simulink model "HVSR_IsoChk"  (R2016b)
settings: Solver=VariableStepAuto  StartTime=0.0  StopTime=10.0  RelTol=1e-3
undefined symbols (not defined in the file or in its folder): bin2dec, enmActv, enmBmsMode, enmCctErr, enmSWSta, HVSR_bIsoResShieldCal, HVSR_bSw1EnaByMnl_C, HVSR_bSw2EnaByMnl_C, HVSR_bSw3EnaByMnl_C, HVSR_bSwEnaByMnl_C, HVSR_bVldEnaByMnl_C, HVSR_cntIsoChkCnfDiag_C, HVSR_cntIsoChkCnfLv1Diag_C, HVSR_cntIsoChkDiag_CW, HVSR_cntPwrDown_C, HVSR_cofPosVoltfilter_C, HVSR_cofResGain_C, HVSR_deltInsRes_C, HVSR_InsResCtrlSw_C, HVSR_kSlopeVal_C, HVSR_numBgnTimeCnt_C, HVSR_numCycleTimeCnt_C, HVSR_numIsoCnst_C, HVSR_numSlopeCnfrm_C, HVSR_ResFirstCtrlSw_C, HVSR_resIsoFaultLvl1Thres_C, HVSR_resIsoFaultLvl2Thres_C, HVSR_ResR1_C, HVSR_ResR2_C, HVSR_ResR3_C, HVSR_resRstnUpLim_C, HVSR_rIsoCnfHysDiag_C, HVSR_rIsoCnfHysLv1Diag_C, HVSR_stBMSModeLvl_C, HVSR_tiChkFilteTime_C, HVSR_tiIsoChkCycl_T, HVSR_tiIsoChkDebounce_C, HVSR_tiIsoVldChkDebounce_C, HVSR_tiTaskTime_C, HVSR_tiVoltDiffThres_C, HVSR_uBattVoltRngHi_C, HVSR_uBattVoltRngLo_C, HVSR_uIsoKVoltThres_C, HVSR_uIsoPosVoltFilter_C, HVSR_uIsoVoltThres_C
libraries: simulink x78
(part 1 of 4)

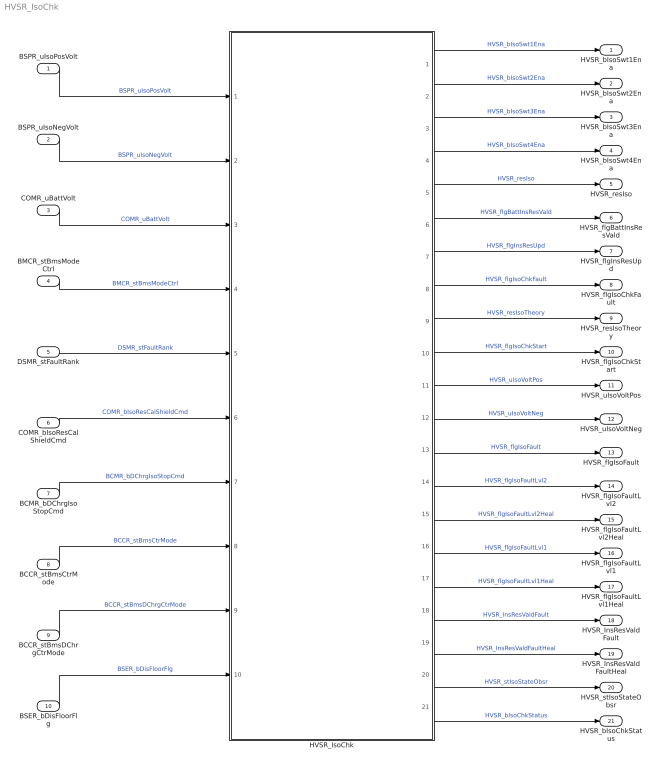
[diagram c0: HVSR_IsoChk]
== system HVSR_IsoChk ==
  BSPR_uIsoPosVolt : Inport  Description=Power battery postive to case voltage
  BSPR_uIsoNegVolt : Inport  Description=Power battery negative to case voltage  Port=2
  COMR_uBattVolt : Inport  Description=Battery pack total voltage  Port=3
  BMCR_stBmsModeCtrl : Inport  Port=4
  DSMR_stFaultRank : Inport  Port=5
  COMR_bIsoResCalShieldCmd : Inport  Port=6
  BCMR_bDChrgIsoStopCmd : Inport  Port=7
  BCCR_stBmsCtrMode : Inport  Port=8
  BCCR_stBmsDChrgCtrMode : Inport  Port=9
  BSER_bDisFloorFlg : Inport  Port=10
  HVSR_IsoChk : Subsystem  Description=Battery pack insulation detection module
  HVSR_bIsoSwt1Ena : Outport  Description=Insulation detection positive relay control command
  HVSR_bIsoSwt2Ena : Outport  Description=Insulation detection positive relay control command  Port=2
  HVSR_bIsoSwt3Ena : Outport  Description=Insulation detection positive relay control command  Port=3
  HVSR_bIsoSwt4Ena : Outport  Description=Insulation detection positive relay control command  Port=4
  HVSR_resIso : Outport  Description=Insulation detection resistance validity flag  Port=5
  HVSR_flgBattInsResVald : Outport  Description=Insulation detection resistance validity flag  Port=6
  HVSR_flgInsResUpd : Outport  Description=Insulation detection resistance pass flag  Port=7
  HVSR_flgIsoChkFault : Outport  Description=Insulation detection resistance pass flag  Port=8
  HVSR_resIsoTheory : Outport  Description=Insulation detection resistance pass flag  Port=9
  HVSR_flgIsoChkStart : Outport  Port=10
  HVSR_uIsoVoltPos : Outport  Port=11
  HVSR_uIsoVoltNeg : Outport  Port=12
  HVSR_flgIsoFault : Outport  Description=Insulation detection resistance pass flag  Port=13
  HVSR_flgIsoFaultLvl2 : Outport  Port=14
  HVSR_flgIsoFaultLvl2Heal : Outport  Port=15
  HVSR_flgIsoFaultLvl1 : Outport  Port=16
  HVSR_flgIsoFaultLvl1Heal : Outport  Port=17
  HVSR_InsResValdFault : Outport  Port=18
  HVSR_InsResValdFaultHeal : Outport  Port=19
  HVSR_stIsoStateObsr : Outport  Port=20
  HVSR_bIsoChkStatus : Outport  Port=21
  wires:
  BSPR_uIsoPosVolt/1 -> HVSR_IsoChk/1(BSPR_uIsoPosVolt)  "BSPR_uIsoPosVolt"
  COMR_uBattVolt/1 -> HVSR_IsoChk/3(BSPR_uBattVolt)  "COMR_uBattVolt"
  HVSR_IsoChk/1(HVSR_bIsoSwt1Ena) -> HVSR_bIsoSwt1Ena/1  "HVSR_bIsoSwt1Ena"
  HVSR_IsoChk/2(HVSR_bIsoSwt2Ena) -> HVSR_bIsoSwt2Ena/1  "HVSR_bIsoSwt2Ena"
  HVSR_IsoChk/3(HVSR_bIsoSwt3Ena) -> HVSR_bIsoSwt3Ena/1  "HVSR_bIsoSwt3Ena"
  HVSR_IsoChk/6(HVSR_flgBattInsResVald) -> HVSR_flgBattInsResVald/1  "HVSR_flgBattInsResVald"
  HVSR_IsoChk/13(HVSR_flgIsoFault) -> HVSR_flgIsoFault/1  "HVSR_flgIsoFault"
  HVSR_IsoChk/5(HVSR_resIso) -> HVSR_resIso/1  "HVSR_resIso"
  HVSR_IsoChk/7(HVSR_flgInsResUpd) -> HVSR_flgInsResUpd/1  "HVSR_flgInsResUpd"
  HVSR_IsoChk/8(HVSR_flgIsoChkFault) -> HVSR_flgIsoChkFault/1  "HVSR_flgIsoChkFault"
  HVSR_IsoChk/9(HVSR_resIsoTheory) -> HVSR_resIsoTheory/1  "HVSR_resIsoTheory"
  HVSR_IsoChk/11(HVSR_uIsoVoltPos) -> HVSR_uIsoVoltPos/1  "HVSR_uIsoVoltPos"
  HVSR_IsoChk/10(HVSR_flgIsoChkStart) -> HVSR_flgIsoChkStart/1  "HVSR_flgIsoChkStart"
  DSMR_stFaultRank/1 -> HVSR_IsoChk/5(DSMR_stFaultRank)  "DSMR_stFaultRank"
  BMCR_stBmsModeCtrl/1 -> HVSR_IsoChk/4(BMCR_stBmsModeCtrl)  "BMCR_stBmsModeCtrl"
  HVSR_IsoChk/14(HVSR_flgIsoFaultLvl2) -> HVSR_flgIsoFaultLvl2/1  "HVSR_flgIsoFaultLvl2"
  HVSR_IsoChk/15(HVSR_flgIsoFaultLvl2Heal) -> HVSR_flgIsoFaultLvl2Heal/1  "HVSR_flgIsoFaultLvl2Heal"
  HVSR_IsoChk/16(HVSR_flgIsoFaultLvl1) -> HVSR_flgIsoFaultLvl1/1  "HVSR_flgIsoFaultLvl1"
  HVSR_IsoChk/17(HVSR_flgIsoFaultLvl1Heal) -> HVSR_flgIsoFaultLvl1Heal/1  "HVSR_flgIsoFaultLvl1Heal"
  HVSR_IsoChk/19(HVSR_InsResValdFaultHeal) -> HVSR_InsResValdFaultHeal/1  "HVSR_InsResValdFaultHeal"
  HVSR_IsoChk/18(HVSR_InsResValdFault) -> HVSR_InsResValdFault/1  "HVSR_InsResValdFault"
  COMR_bIsoResCalShieldCmd/1 -> HVSR_IsoChk/6(COMR_bIsoResCalShieldCmd)  "COMR_bIsoResCalShieldCmd"
  BCMR_bDChrgIsoStopCmd/1 -> HVSR_IsoChk/7(BCMR_bDChrgIsoStopCmd)  "BCMR_bDChrgIsoStopCmd"
  HVSR_IsoChk/20(HVSR_stIsoStateObsr) -> HVSR_stIsoStateObsr/1  "HVSR_stIsoStateObsr"
  HVSR_IsoChk/21(HVSR_bIsoChkStatus) -> HVSR_bIsoChkStatus/1  "HVSR_bIsoChkStatus"
  BSPR_uIsoNegVolt/1 -> HVSR_IsoChk/2(BSPR_uIsoNegVolt)  "BSPR_uIsoNegVolt"
  HVSR_IsoChk/4(HVSR_bIsoSwt4Ena) -> HVSR_bIsoSwt4Ena/1  "HVSR_bIsoSwt4Ena"
  HVSR_IsoChk/12(HVSR_uIsoVoltNeg) -> HVSR_uIsoVoltNeg/1  "HVSR_uIsoVoltNeg"
  BCCR_stBmsCtrMode/1 -> HVSR_IsoChk/8(BCCR_stBmsCtrMode)  "BCCR_stBmsCtrMode"
  BCCR_stBmsDChrgCtrMode/1 -> HVSR_IsoChk/9(BCCR_stBmsDChrgCtrMode)  "BCCR_stBmsDChrgCtrMode"
  BSER_bDisFloorFlg/1 -> HVSR_IsoChk/10(BSER_bDisFloorFlg)  "BSER_bDisFloorFlg"

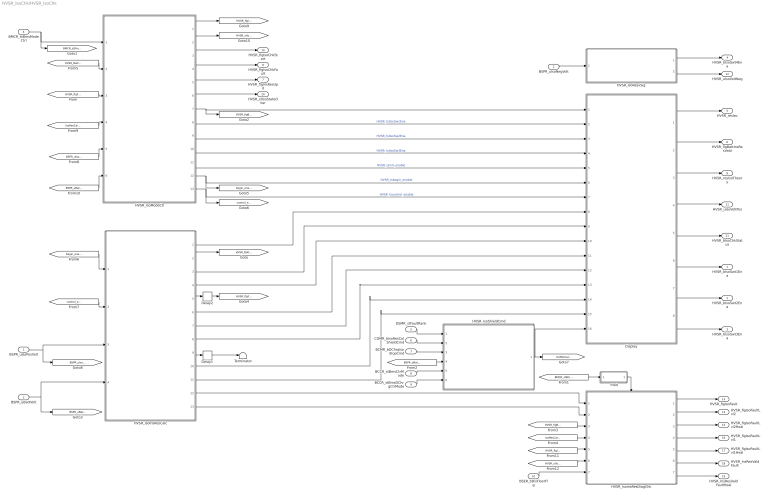
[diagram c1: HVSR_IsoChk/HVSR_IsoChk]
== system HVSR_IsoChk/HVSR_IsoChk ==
  BSPR_uIsoPosVolt : Inport
  BSPR_uIsoNegVolt : Inport  Description=Power battery negative to case voltage  Port=2
  BSPR_uBattVolt : Inport  Port=3
  BMCR_stBmsModeCtrl : Inport  Port=4
  DSMR_stFaultRank : Inport  Port=5
  COMR_bIsoResCalShieldCmd : Inport  Port=6
  BCMR_bDChrgIsoStopCmd : Inport  Port=7
  BCCR_stBmsCtrMode : Inport  Port=8
  BCCR_stBmsDChrgCtrMode : Inport  Port=9
  BSER_bDisFloorFlg : Inport  Port=10
  Delay1 : Delay  DelayLength=1  InitialCondition=0
  Delay2 : Delay  DelayLength=1  InitialCondition=0
  Display : Subsystem  Description=Battery pack insulation detection Display module
  HVSR_IsoInsResCalc : Subsystem  Description=Battery pack insulation detection Control module
  HVSR_IsoInsResDiagChk : Subsystem
  HVSR_IsoModeCtr : Subsystem
  HVSR_IsoResvSig : Subsystem
  HVSR_IsoShieldCmd : Subsystem
  Terminator : Terminator
  mod : Subsystem
  HVSR_bIsoSwt1Ena : Outport
  HVSR_bIsoSwt2Ena : Outport  Port=2
  HVSR_bIsoSwt3Ena : Outport  Port=3
  HVSR_bIsoSwt4Ena : Outport  Port=4
  HVSR_resIso : Outport  Port=5
  HVSR_flgBattInsResVald : Outport  Port=6
  HVSR_flgInsResUpd : Outport  Port=7
  HVSR_flgIsoChkFault : Outport  Port=8
  HVSR_resIsoTheory : Outport  Port=9
  HVSR_flgIsoChkStart : Outport  Port=10
  HVSR_uIsoVoltPos : Outport  Port=11
  HVSR_uIsoVoltNeg : Outport  Port=12
  HVSR_flgIsoFault : Outport  Port=13
  HVSR_flgIsoFaultLvl2 : Outport  Port=14
  HVSR_flgIsoFaultLvl2Heal : Outport  Port=15
  HVSR_flgIsoFaultLvl1 : Outport  Port=16
  HVSR_flgIsoFaultLvl1Heal : Outport  Port=17
  HVSR_InsResValdFault : Outport  Port=18
  HVSR_InsResValdFaultHeal : Outport  Port=19
  HVSR_stIsoStateObsr : Outport  Port=20
  HVSR_bIsoChkStatus : Outport  Port=21
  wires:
  BSPR_uBattVolt/1 -> HVSR_IsoInsResCalc/4(BSPR_uBattVolt), [BSPR_uBattVolt]
  Display/1(HVSR_resIso) -> HVSR_resIso/1
  Display/2(HVSR_flgBattInsResVald) -> HVSR_flgBattInsResVald/1
  Display/3(HVSR_resIsoTheory) -> HVSR_resIsoTheory/1
  Display/4(HVSR_uIsoVoltPos) -> HVSR_uIsoVoltPos/1
  HVSR_IsoInsResCalc/2(HVSR_BattInsResVald) -> [HVSR_BattInsResVald]
  HVSR_IsoInsResDiagChk/1(HVSR_flgIsoFault) -> HVSR_flgIsoFault/1
  HVSR_IsoInsResDiagChk/2(HVSR_flgIsoFaultLvl2) -> HVSR_flgIsoFaultLvl2/1
  HVSR_IsoInsResDiagChk/3(HVSR_flgIsoFaultLvl2Heal) -> HVSR_flgIsoFaultLvl2Heal/1
  HVSR_IsoInsResDiagChk/4(HVSR_flgIsoFaultLvl1) -> HVSR_flgIsoFaultLvl1/1
  HVSR_IsoInsResDiagChk/5(HVSR_flgIsoFaultLvl1Heal) -> HVSR_flgIsoFaultLvl1Heal/1
  BSPR_uIsoPosVolt/1 -> HVSR_IsoInsResCalc/3(BSPR_uIsoPosVolt), [BSPR_uIsoNegVolt]
  HVSR_IsoInsResCalc/5(HVSR_flgFrstRsVlotVld) -> Delay2/1
  Delay2/1 -> [HVSR_flgFrstRsVlotVld]
  mod/1(Out1) -> HVSR_IsoInsResDiagChk/Enable
  HVSR_IsoInsResDiagChk/6(HVSR_InsResValdFault) -> HVSR_InsResValdFault/1
  HVSR_IsoInsResDiagChk/7(HVSR_InsResValdFaultHeal) -> HVSR_InsResValdFaultHeal/1
  Display/5(HVSR_bIsoChkStatus) -> HVSR_bIsoChkStatus/1
  DSMR_stFaultRank/1 -> HVSR_IsoShieldCmd/1(DSMR_stFaultRank)
  COMR_bIsoResCalShieldCmd/1 -> HVSR_IsoShieldCmd/2(COMR_bIsoResCalShieldCmd)
  BCMR_bDChrgIsoStopCmd/1 -> HVSR_IsoShieldCmd/3(BCMR_bDChrgIsoStopCmd)
  HVSR_IsoModeCtr/3(HVSR_flgIsoChkStart) -> HVSR_flgIsoChkStart/1
  HVSR_IsoModeCtr/4(HVSR_flgIsoChkFault) -> HVSR_flgIsoChkFault/1
  HVSR_IsoModeCtr/5(HVSR_flgInsResUpd) -> HVSR_flgInsResUpd/1
  HVSR_IsoModeCtr/6(HVSR_stIsoStateObsr) -> HVSR_stIsoStateObsr/1
  [HVSR_BattInsResVald] -> HVSR_IsoModeCtr/2(HVSR_BattInsResVald)
  [HVSR_flgFrstRsVlotVld] -> HVSR_IsoModeCtr/3(HVSR_flgFrstRsVlotVld)
  [IsoResCalShieldCmd] -> HVSR_IsoModeCtr/4(IsoResCalShieldCmd)
  BSPR_uIsoNegVolt/1 -> HVSR_IsoResvSig/1(BSPR_uIsoNegVolt)
  HVSR_IsoResvSig/1(HVSR_bIsoSwt4Ena) -> HVSR_bIsoSwt4Ena/1
  HVSR_IsoResvSig/2(HVSR_uIsoVoltNeg) -> HVSR_uIsoVoltNeg/1
  HVSR_IsoModeCtr/12(begin_enable) -> [begin_enable], Display/6(begin_enable)  "HVSR_tsbegin_enable"
  HVSR_IsoInsResCalc/1(HVSR_IsoBattInsRes) -> Display/8(HVSR_IsoBattInsRes)
  HVSR_IsoInsResCalc/3(HVSR_IsoInsResTheory) -> Display/9(HVSR_IsoResThry)
  HVSR_IsoInsResCalc/12(flgIsoFaultLvl1) -> HVSR_IsoInsResDiagChk/1(flgIsoFaultLvl1)
  HVSR_IsoInsResCalc/13(flgIsoFaultLvl2) -> HVSR_IsoInsResDiagChk/2(flgIsoFaultLvl2)
  Display/6(HVSR_bIsoSwt1Ena) -> HVSR_bIsoSwt1Ena/1
  Display/8(HVSR_bIsoSwt3Ena) -> HVSR_bIsoSwt3Ena/1
  HVSR_IsoModeCtr/11(init_enable) -> Display/5(init_enable)  "HVSR_tsinit_enable"
  [BMCR_stBmsModeCtrl] -> mod/1(In1)
  [HVSR_flgBattInsResVld] -> HVSR_IsoInsResDiagChk/3(flgBattInsResVald)
  HVSR_IsoModeCtr/7(HVSR_flgBattInsResVld) -> [HVSR_flgBattInsResVld], Display/1(HVSR_IsoResVald)
  HVSR_IsoModeCtr/8(HVSR_IsoSwt1Ena) -> Display/2(bIsoSwt1Ena)  "HVSR_tsIIsoSw1Ena"
  HVSR_IsoModeCtr/9(HVSR_IsoSwt2Ena) -> Display/3(bIsoSwt2Ena)  "HVSR_tsIIsoSw2Ena"
  HVSR_IsoModeCtr/10(HVSR_IsoSwt3Ena) -> Display/4(bIsoSwt3Ena)  "HVSR_tsIIsoSw3Ena"
  [IsoResCalShieldCmd] -> HVSR_IsoInsResDiagChk/4(IsoResCalShield)
  HVSR_IsoShieldCmd/1(HVSR_IsoChieldCmd) -> Display/16(HVSR_IsoChieldCmd), [IsoResCalShieldCmd]
  HVSR_IsoInsResCalc/4("HVSR_uIsoFrstRsVolt ") -> Display/10(HVSR_uIsoFrstRsVolt)
  HVSR_IsoInsResCalc/8(HVSR_uIsoScndRsVolt) -> Display/13(HVSR_uIsoScndRsVolt)
  HVSR_IsoInsResCalc/9(HVSR_flgScndRsVlotVld) -> Delay1/1
  Delay1/1 -> Terminator/1
  HVSR_IsoModeCtr/13(control_enable) -> [control_enable], Display/7(control_enable)  "HVSR_tscontrol_enable"
  HVSR_IsoInsResCalc/7(HVSR_numIsoFrstVal) -> Display/12(HVSR_numIsoFrstVal)
  HVSR_IsoInsResCalc/6(HVSR_uFrstRsVlot) -> Display/11(HVSR_uFrstRsVlot)
  HVSR_IsoInsResCalc/11(HVSR_numIsoScndVal) -> Display/15(HVSR_numIsoScndVal)
  HVSR_IsoInsResCalc/10(HVSR_uScndRsVlot) -> Display/14(HVSR_uScndRsVlot)
  BMCR_stBmsModeCtrl/1 -> [BMCR_stBmsModeCtrl], HVSR_IsoModeCtr/1(BMCR_stBmsModeCtrl)
  Display/7(HVSR_bIsoSwt2Ena) -> HVSR_bIsoSwt2Ena/1
  [begin_enable] -> HVSR_IsoInsResCalc/1(begin_enable)
  [control_enable] -> HVSR_IsoInsResCalc/2(control_enable)
  [BSPR_uBattVolt] -> HVSR_IsoShieldCmd/4(BSPR_uBattVolt)
  BCCR_stBmsCtrMode/1 -> HVSR_IsoShieldCmd/5(BCCR_stBmsCtrMode)
  BCCR_stBmsDChrgCtrMode/1 -> HVSR_IsoShieldCmd/6(BCCR_stBmsDChrgCtrMode)
  [BSPR_uIsoNegVolt] -> HVSR_IsoModeCtr/5(BSPR_uIsoNegVolt)
  [BSPR_uBattVolt] -> HVSR_IsoModeCtr/6(BSPR_uBattVolt)
  HVSR_IsoModeCtr/1(HVSR_flgIsoCctChkOK) -> [HVSR_flgIsoCctChkOK]
  HVSR_IsoModeCtr/2(HVSR_stIsoCctChkErr) -> [HVSR_stIsoCctChkErr]
  [HVSR_flgIsoCctChkOK] -> HVSR_IsoInsResDiagChk/5(HVSR_flgIsoCctChkOK)
  [HVSR_stIsoCctChkErr] -> HVSR_IsoInsResDiagChk/6(HVSR_stIsoCctChkE rr)
  BSER_bDisFloorFlg/1 -> HVSR_IsoInsResDiagChk/7(BSER_bDisFloorFlg)

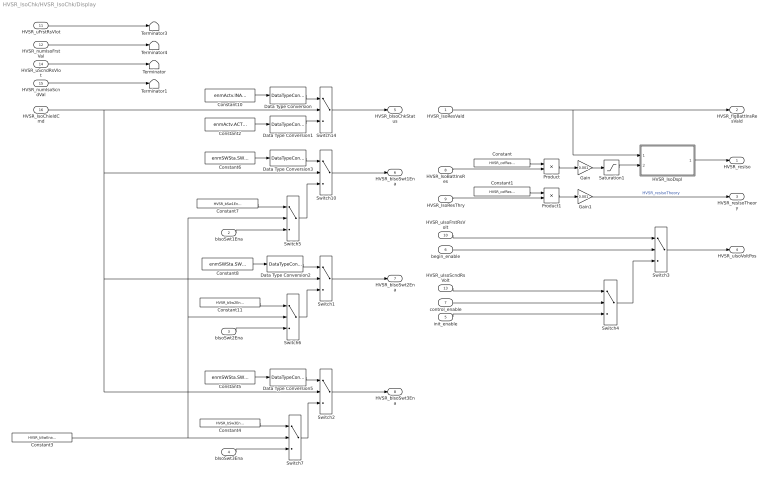
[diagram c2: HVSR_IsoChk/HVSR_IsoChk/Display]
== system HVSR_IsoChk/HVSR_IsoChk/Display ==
  HVSR_IsoResVald : Inport
  bIsoSwt1Ena : Inport  Port=2
  bIsoSwt2Ena : Inport  Port=3
  bIsoSwt3Ena : Inport  Port=4
  init_enable : Inport  Port=5
  begin_enable : Inport  Port=6
  control_enable : Inport  Port=7
  HVSR_IsoBattInsRes : Inport  Port=8
  HVSR_IsoResThry : Inport  Port=9
  HVSR_uIsoFrstRsVolt : Inport  Port=10
  HVSR_uFrstRsVlot : Inport  Port=11
  HVSR_numIsoFrstVal : Inport  Port=12
  HVSR_uIsoScndRsVolt : Inport  Port=13
  HVSR_uScndRsVlot : Inport  Port=14
  HVSR_numIsoScndVal : Inport  Port=15
  HVSR_IsoChieldCmd : Inport  Port=16
  Constant : Constant  Value=HVSR_cofResGain_C
  Constant1 : Constant  Value=HVSR_cofResGain_C
  Constant10 : Constant  Value=enmActv.INACTIVE  OutDataTypeStr=Enum: enmActv
  Constant11 : Constant  Value=HVSR_bSw2EnaByMnl_C
  Constant2 : Constant  Value=enmActv.ACTIVE  OutDataTypeStr=Enum: enmActv
  Constant3 : Constant  Value=HVSR_bSwEnaByMnl_C
  Constant4 : Constant  Value=HVSR_bSw3EnaByMnl_C
  Constant5 : Constant  Value=enmSWSta.SWOFF  OutDataTypeStr=Enum: enmSWSta
  Constant6 : Constant  Value=enmSWSta.SWOFF  OutDataTypeStr=Enum: enmSWSta
  Constant7 : Constant  Value=HVSR_bSw1EnaByMnl_C
  Constant8 : Constant  Value=enmSWSta.SWOFF  OutDataTypeStr=Enum: enmSWSta
  Data Type Conversion{,1..3,5} (5 alike) : DataTypeConversion  OutDataTypeStr=boolean
  Gain : Gain  Gain=0.001
  Gain1 : Gain  Gain=0.001
  HVSR_IsoDspl : Subsystem
  Product : Product
  Product1 : Product
  Saturation1 : Saturate  UpperLimit=HVSR_resRstnUpLim_C  LowerLimit=0
  Switch{1..7,10,14} (9 alike) : Switch  Criteria=u2 ~= 0
  Terminator{,1,3..4} (4 alike) : Terminator
  HVSR_resIso : Outport
  HVSR_flgBattInsResVald : Outport  Port=2
  HVSR_resIsoTheory : Outport  Port=3
  HVSR_uIsoVoltPos : Outport  Port=4
  HVSR_bIsoChkStatus : Outport  Port=5
  HVSR_bIsoSwt1Ena : Outport  Port=6
  HVSR_bIsoSwt2Ena : Outport  Port=7
  HVSR_bIsoSwt3Ena : Outport  Port=8
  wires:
  HVSR_IsoResVald/1 -> HVSR_IsoDspl/1(In1), HVSR_flgBattInsResVald/1
  Gain/1 -> Saturation1/1
  Gain1/1 -> HVSR_resIsoTheory/1  "HVSR_resIsoTheory"
  Product/1 -> Gain/1
  HVSR_IsoBattInsRes/1 -> Product/2
  Constant/1 -> Product/1
  Product1/1 -> Gain1/1
  HVSR_IsoResThry/1 -> Product1/2
  Constant1/1 -> Product1/1
  Saturation1/1 -> HVSR_IsoDspl/2(In3)
  HVSR_IsoDspl/1(HVSR_resIso) -> HVSR_resIso/1
  Switch14/1 -> HVSR_bIsoChkStatus/1
  Constant10/1 -> Data Type Conversion/1
  Data Type Conversion/1 -> Switch14/1
  Constant2/1 -> Data Type Conversion1/1
  Data Type Conversion1/1 -> Switch14/3
  Switch10/1 -> HVSR_bIsoSwt1Ena/1
  Data Type Conversion3/1 -> Switch10/1
  bIsoSwt1Ena/1 -> Switch5/3
  Constant6/1 -> Data Type Conversion3/1
  Switch1/1 -> HVSR_bIsoSwt2Ena/1
  Data Type Conversion2/1 -> Switch1/1
  HVSR_IsoChieldCmd/1 -> Switch10/2, Switch2/2, Switch1/2, Switch14/2
  Switch2/1 -> HVSR_bIsoSwt3Ena/1
  Data Type Conversion5/1 -> Switch2/1
  bIsoSwt3Ena/1 -> Switch7/3
  Constant5/1 -> Data Type Conversion5/1
  HVSR_uScndRsVlot/1 -> Terminator/1
  HVSR_uFrstRsVlot/1 -> Terminator3/1
  HVSR_numIsoScndVal/1 -> Terminator1/1
  HVSR_numIsoFrstVal/1 -> Terminator4/1
  begin_enable/1 -> Switch3/2
  HVSR_uIsoFrstRsVolt/1 -> Switch3/1
  Switch4/1 -> Switch3/3
  control_enable/1 -> Switch4/2
  Switch3/1 -> HVSR_uIsoVoltPos/1
  HVSR_uIsoScndRsVolt/1 -> Switch4/1
  init_enable/1 -> Switch4/3
  Switch5/1 -> Switch10/3
  Constant7/1 -> Switch5/1
  Constant8/1 -> Data Type Conversion2/1
  bIsoSwt2Ena/1 -> Switch6/3
  Constant3/1 -> Switch5/2, Switch6/2, Switch7/2
  Constant11/1 -> Switch6/1
  Switch6/1 -> Switch1/3
  Constant4/1 -> Switch7/1
  Switch7/1 -> Switch2/3

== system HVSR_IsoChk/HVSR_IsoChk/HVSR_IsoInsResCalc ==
  begin_enable : Inport
  control_enable : Inport  Port=2
  BSPR_uIsoPosVolt : Inport  Port=3
  BSPR_uBattVolt : Inport  Port=4
  Constant : Constant  OutDataTypeStr=boolean
  HVSR_IsoInsResAlg : Subsystem  Description=Battery pack insulation detection Algorithm module
  HVSR_IsoInsResDiag : Subsystem  Description=Battery pack insulation detection JudgeBlock module
  HVSR_IsoVoltFilter : Subsystem
  HVSR_IsoBattInsRes : Outport  InitialOutput=0
  HVSR_BattInsResVald : Outport  Port=2
  HVSR_IsoInsResTheory : Outport  Port=3  InitialOutput=0
  "HVSR_uIsoFrstRsVolt " : Outport  Port=4  InitialOutput=0.
  HVSR_flgFrstRsVlotVld : Outport  Port=5  InitialOutput=0.
  HVSR_uFrstRsVlot : Outport  Port=6  InitialOutput=0.
  HVSR_numIsoFrstVal : Outport  Port=7  InitialOutput=0.
  HVSR_uIsoScndRsVolt : Outport  Port=8  InitialOutput=0.
  HVSR_flgScndRsVlotVld : Outport  Port=9  InitialOutput=0.
  HVSR_uScndRsVlot : Outport  Port=10  InitialOutput=0.
  HVSR_numIsoScndVal : Outport  Port=11  InitialOutput=0.
  flgIsoFaultLvl1 : Outport  Port=12
  flgIsoFaultLvl2 : Outport  Port=13
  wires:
  BSPR_uBattVolt/1 -> HVSR_IsoInsResAlg/5(BSPR_uBattVolt)
  BSPR_uIsoPosVolt/1 -> HVSR_IsoVoltFilter/1(BSPR_uIsoPosVolt)
  HVSR_IsoInsResAlg/1(HVSR_IsoBattInsRes) -> HVSR_IsoBattInsRes/1, HVSR_IsoInsResDiag/1(HVSR_IsoBattInsRes)
  HVSR_IsoInsResAlg/2(HVSR_flgInsResVld) -> HVSR_BattInsResVald/1  "HVSR_BattInsResVald"
  HVSR_IsoInsResAlg/3(HVSR_IsoInsResTheory) -> HVSR_IsoInsResTheory/1
  HVSR_IsoInsResAlg/4(HVSR_uIsoFrstRsVolt) -> "HVSR_uIsoFrstRsVolt "/1
  HVSR_IsoInsResDiag/2(BattIsolationFaultLvl1) -> flgIsoFaultLvl1/1
  HVSR_IsoInsResDiag/1(BattIsolationFaultLvl2) -> flgIsoFaultLvl2/1
  begin_enable/1 -> HVSR_IsoInsResAlg/1(begin_enable)
  control_enable/1 -> HVSR_IsoInsResAlg/2(control_enable)
  HVSR_IsoVoltFilter/1(HVSR_uIsoRsVolt) -> HVSR_IsoInsResAlg/4(HVSR_uIsoRsVolt)
  Constant/1 -> HVSR_IsoInsResAlg/3(IsoSwtLastTEna)
  HVSR_IsoInsResAlg/5(HVSR_flgFrstRsVlotVld) -> HVSR_flgFrstRsVlotVld/1
  HVSR_IsoInsResAlg/6(HVSR_uFrstRsVlot) -> HVSR_uFrstRsVlot/1
  HVSR_IsoInsResAlg/7(HVSR_numIsoFrstVal) -> HVSR_numIsoFrstVal/1
  HVSR_IsoInsResAlg/8(HVSR_uIsoScndRsVolt) -> HVSR_uIsoScndRsVolt/1
  HVSR_IsoInsResAlg/10(HVSR_uScndRsVlot) -> HVSR_uScndRsVlot/1
  HVSR_IsoInsResAlg/9(HVSR_flgScndRsVlotVld) -> HVSR_flgScndRsVlotVld/1
  HVSR_IsoInsResAlg/11(HVSR_numIsoScndVal) -> HVSR_numIsoScndVal/1

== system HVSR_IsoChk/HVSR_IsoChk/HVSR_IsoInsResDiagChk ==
  flgIsoFaultLvl1 : Inport
  flgIsoFaultLvl2 : Inport  Port=2
  flgBattInsResVald : Inport  Port=3
  IsoResCalShield : Inport  Port=4
  HVSR_flgIsoCctChkOK : Inport  Port=5
  HVSR_stIsoCctChkE rr : Inport  Port=6
  BSER_bDisFloorFlg : Inport  Port=7
  Enable : EnablePort
  HVSR_IsoErrHeal : Subsystem
  HVSR_IsoFaultHeal : Subsystem
  HVSR_flgIsoFault : Outport
  HVSR_flgIsoFaultLvl2 : Outport  Port=2
  HVSR_flgIsoFaultLvl2Heal : Outport  Port=3
  HVSR_flgIsoFaultLvl1 : Outport  Port=4
  HVSR_flgIsoFaultLvl1Heal : Outport  Port=5
  HVSR_InsResValdFault : Outport  Port=6
  HVSR_InsResValdFaultHeal : Outport  Port=7
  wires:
  HVSR_IsoFaultHeal/1(" HVSR_flgIsoFault") -> HVSR_flgIsoFault/1
  HVSR_IsoFaultHeal/7(DFC_InsResValdFaultHeal) -> HVSR_InsResValdFaultHeal/1
  HVSR_IsoFaultHeal/2(DFC_flgIsoFaultLvl2) -> HVSR_flgIsoFaultLvl2/1
  HVSR_IsoFaultHeal/3(DFC_flgIsoFaultLvl2Heal) -> HVSR_flgIsoFaultLvl2Heal/1
  HVSR_IsoFaultHeal/6(DFC_InsResValdFault) -> HVSR_InsResValdFault/1
  HVSR_IsoFaultHeal/4(DFC_flgIsoFaultLvl1) -> HVSR_flgIsoFaultLvl1/1
  HVSR_IsoFaultHeal/5(DFC_flgIsoFaultLvl1Heal) -> HVSR_flgIsoFaultLvl1Heal/1
  flgIsoFaultLvl2/1 -> HVSR_IsoErrHeal/1(flgIsoFaultLvl2)
  flgIsoFaultLvl1/1 -> HVSR_IsoErrHeal/2(flgIsoFaultLvl1)
  flgBattInsResVald/1 -> HVSR_IsoErrHeal/3(flgBattInsResVald)
  IsoResCalShield/1 -> HVSR_IsoErrHeal/4(IsoResCalShield)
  HVSR_IsoErrHeal/1(HVSR_flgIsoFaultLvl2) -> HVSR_IsoFaultHeal/1(HVSR_flgIsoFaultLvl2)
  HVSR_IsoErrHeal/2(HVSR_flgIsoFaultLvl2Heal) -> HVSR_IsoFaultHeal/2(HVSR_flgIsoFaultLvl2Heal)
  HVSR_IsoErrHeal/3(HVSR_flgIsoFaultLvl1) -> HVSR_IsoFaultHeal/3(HVSR_flgIsoFaultLvl1)
  HVSR_IsoErrHeal/4(HVSR_flgIsoFaultLvl1Heal) -> HVSR_IsoFaultHeal/4(HVSR_flgIsoFaultLvl1Heal)
  HVSR_IsoErrHeal/5(HVSR_InsResValdFault) -> HVSR_IsoFaultHeal/5(HVSR_InsResValdFault)
  HVSR_IsoErrHeal/6(HVSR_InsResValdFaultHeal) -> HVSR_IsoFaultHeal/6(HVSR_InsResValdFaultHeal)
  HVSR_stIsoCctChkE rr/1 -> HVSR_IsoFaultHeal/8(HVSR_stIsoCctChkErr)
  HVSR_flgIsoCctChkOK/1 -> HVSR_IsoFaultHeal/7(HVSR_flgIsoCctChkOK)
  BSER_bDisFloorFlg/1 -> HVSR_IsoErrHeal/5(BSER_bDisFloorFlg)

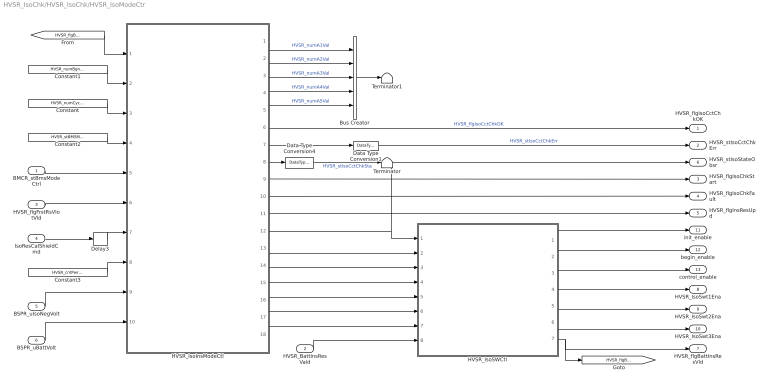
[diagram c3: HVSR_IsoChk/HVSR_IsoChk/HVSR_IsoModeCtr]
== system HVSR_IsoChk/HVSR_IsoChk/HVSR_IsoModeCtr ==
  BMCR_stBmsModeCtrl : Inport
  HVSR_BattInsResVald : Inport  Port=2
  HVSR_flgFrstRsVlotVld : Inport  Port=3
  IsoResCalShieldCmd : Inport  Port=4
  BSPR_uIsoNegVolt : Inport  Port=5
  BSPR_uBattVolt : Inport  Port=6
  Bus Creator : BusCreator  Inputs=5
  Constant : Constant  Value=HVSR_numCycleTimeCnt_C
  Constant1 : Constant  Value=HVSR_numBgnTimeCnt_C
  Constant2 : Constant  Value=HVSR_stBMSModeLvl_C
  Constant3 : Constant  Value=HVSR_cntPwrDown_C
  Data Type Conversion1 : DataTypeConversion  OutDataTypeStr=uint8
  Data Type Conversion4 : DataTypeConversion  OutDataTypeStr=uint8
  Delay3 : Delay  DelayLength=1  InitialCondition=0
  HVSR_IsoInsModeCtl : Stateflow chart  Description=Battery pack insulation detection Sateflow Mode  TreatAsAtomicUnit=on
  HVSR_IsoSWCtl : Subsystem
  Terminator : Terminator
  Terminator1 : Terminator
  HVSR_flgIsoCctChkOK : Outport
  HVSR_stIsoCctChkErr : Outport  Port=2
  HVSR_flgIsoChkStart : Outport  Port=3
  HVSR_flgIsoChkFault : Outport  Port=4
  HVSR_flgInsResUpd : Outport  Port=5
  HVSR_stIsoStateObsr : Outport  Port=6
  HVSR_flgBattInsResVld : Outport  Port=7
  HVSR_IsoSwt1Ena : Outport  Port=8
  HVSR_IsoSwt2Ena : Outport  Port=9
  HVSR_IsoSwt3Ena : Outport  Port=10
  init_enable : Outport  Port=11
  begin_enable : Outport  Port=12
  control_enable : Outport  Port=13
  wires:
  HVSR_IsoInsModeCtl/11(HVSR_flgInsResUpd) -> HVSR_flgInsResUpd/1
  [HVSR_flgBattInsResVld] -> HVSR_IsoInsModeCtl/1(flgResVald)
  BMCR_stBmsModeCtrl/1 -> HVSR_IsoInsModeCtl/5(BMCR_stBmsModeCtrl)
  HVSR_IsoInsModeCtl/9(HVSR_flgIsoChkStart) -> HVSR_flgIsoChkStart/1
  Constant1/1 -> HVSR_IsoInsModeCtl/2(HVSR_BgTi_C)
  Constant/1 -> HVSR_IsoInsModeCtl/3(HVSR_CycleTi_C)
  Constant2/1 -> HVSR_IsoInsModeCtl/4(HVSR_ModLvl_C)
  HVSR_flgFrstRsVlotVld/1 -> HVSR_IsoInsModeCtl/6(HVSR_flgFrstRsVlotVld)
  HVSR_IsoInsModeCtl/10(HVSR_flgIsoChkFault) -> HVSR_flgIsoChkFault/1
  IsoResCalShieldCmd/1 -> Delay3/1
  Delay3/1 -> HVSR_IsoInsModeCtl/7(IsoResCalShieldCmd)
  HVSR_IsoInsModeCtl/12(HVSR_stIsoStateObsr) -> HVSR_IsoSWCtl/1(HVSR_stIsoStateObsr), HVSR_stIsoStateObsr/1
  HVSR_IsoInsModeCtl/15(begin_enable) -> HVSR_IsoSWCtl/4(HVSR_IsoBeginSta)
  HVSR_IsoInsModeCtl/14(init_enable) -> HVSR_IsoSWCtl/3(HVSR_IsoInitialSta)
  HVSR_IsoInsModeCtl/13(control_enable) -> HVSR_IsoSWCtl/2(HVSR_IsoControlSta)
  HVSR_BattInsResVald/1 -> HVSR_IsoSWCtl/8(HVSR_BattInsResVald)
  HVSR_IsoSWCtl/4(HVSR_IsoSwt1Ena) -> HVSR_IsoSwt1Ena/1
  HVSR_IsoSWCtl/5(HVSR_IsoSwt2Ena) -> HVSR_IsoSwt2Ena/1
  HVSR_IsoSWCtl/6(HVSR_IsoSwt3Ena) -> HVSR_IsoSwt3Ena/1
  HVSR_IsoSWCtl/7(HVSR_flgBattInsResVld) -> HVSR_flgBattInsResVld/1, [HVSR_flgBattInsResVld]
  HVSR_IsoSWCtl/1(init_enable) -> init_enable/1
  HVSR_IsoSWCtl/2(begin_enable) -> begin_enable/1
  HVSR_IsoSWCtl/3(control_enable) -> control_enable/1
  Constant3/1 -> HVSR_IsoInsModeCtl/8(HVSR_cntPwrDown_C)
  BSPR_uIsoNegVolt/1 -> HVSR_IsoInsModeCtl/9(BSPR_uIsoNegVolt)
  BSPR_uBattVolt/1 -> HVSR_IsoInsModeCtl/10(BSPR_uBattVolt)
  HVSR_IsoInsModeCtl/16(HVSR_bIsoChkSW1Sta) -> HVSR_IsoSWCtl/5(HVSR_bIsoChkSW1Sta)
  HVSR_IsoInsModeCtl/17(HVSR_bIsoChkSW2Sta) -> HVSR_IsoSWCtl/6(HVSR_bIsoChkSW2Sta)
  HVSR_IsoInsModeCtl/18(HVSR_bIsoChkSW3Sta) -> HVSR_IsoSWCtl/7(HVSR_bIsoChkSW3Sta)
  HVSR_IsoInsModeCtl/8(HVSR_stIsoCctChkSta) -> Data Type Conversion4/1
  Data Type Conversion4/1 -> Terminator/1  "HVSR_stIsoCctChkSta"
  HVSR_IsoInsModeCtl/6(HVSR_flgIsoCctChkOK) -> HVSR_flgIsoCctChkOK/1  "HVSR_flgIsoCctChkOK"
  HVSR_IsoInsModeCtl/7(HVSR_stIsoCctChkErr) -> Data Type Conversion1/1
  HVSR_IsoInsModeCtl/1(HVSR_numA1Val) -> Bus Creator/1  "HVSR_numA1Val"
  HVSR_IsoInsModeCtl/2(HVSR_numA2Val) -> Bus Creator/2  "HVSR_numA2Val"
  HVSR_IsoInsModeCtl/3(HVSR_numA3Val) -> Bus Creator/3  "HVSR_numA3Val"
  HVSR_IsoInsModeCtl/4(HVSR_numA4Val) -> Bus Creator/4  "HVSR_numA4Val"
  HVSR_IsoInsModeCtl/5(HVSR_numA5Val) -> Bus Creator/5  "HVSR_numA5Val"
  Bus Creator/1 -> Terminator1/1
  Data Type Conversion1/1 -> HVSR_stIsoCctChkErr/1  "HVSR_stIsoCctChkErr"

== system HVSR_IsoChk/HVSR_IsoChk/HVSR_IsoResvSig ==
  BSPR_uIsoNegVolt : Inport  Description=Power battery negative to case voltage
  Constant : Constant  Value=enmSWSta.SWOFF  OutDataTypeStr=Enum: enmSWSta  SampleTime=-1
  Constant1 : Constant  Value=0  OutDataTypeStr=single  SampleTime=-1
  Data Type Conversion : DataTypeConversion  OutDataTypeStr=boolean
  Data Type Conversion1 : DataTypeConversion  OutDataTypeStr=single
  Terminator : Terminator
  HVSR_bIsoSwt4Ena : Outport
  HVSR_uIsoVoltNeg : Outport  Port=2
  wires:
  BSPR_uIsoNegVolt/1 -> Terminator/1
  Data Type Conversion/1 -> HVSR_bIsoSwt4Ena/1
  Data Type Conversion1/1 -> HVSR_uIsoVoltNeg/1
  Constant1/1 -> Data Type Conversion1/1
  Constant/1 -> Data Type Conversion/1

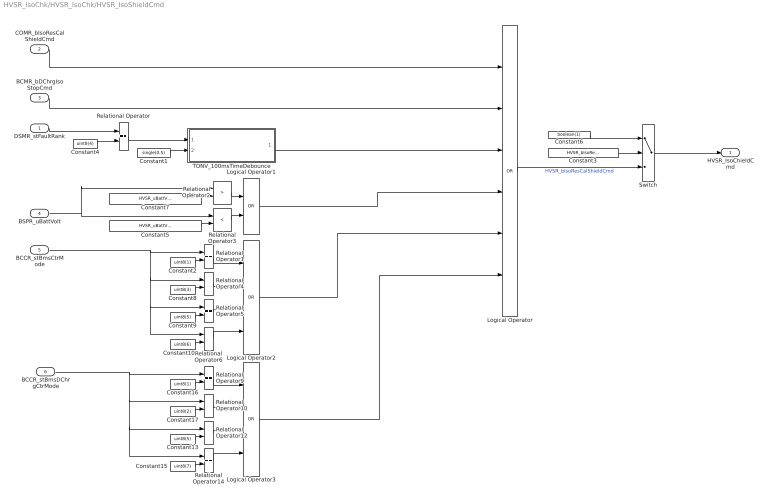
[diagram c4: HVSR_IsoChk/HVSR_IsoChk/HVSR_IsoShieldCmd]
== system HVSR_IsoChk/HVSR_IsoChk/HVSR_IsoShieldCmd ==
  DSMR_stFaultRank : Inport
  COMR_bIsoResCalShieldCmd : Inport  Port=2
  BCMR_bDChrgIsoStopCmd : Inport  Port=3
  BSPR_uBattVolt : Inport  Port=4
  BCCR_stBmsCtrMode : Inport  Port=5
  BCCR_stBmsDChrgCtrMode : Inport  Port=6
  Constant1 : Constant  Value=single(0.5)
  Constant10 : Constant  Value=uint8(6)
  Constant13 : Constant  Value=uint8(5)
  Constant15 : Constant  Value=uint8(7)
  Constant16 : Constant  Value=uint8(1)
  Constant17 : Constant  Value=uint8(2)
  Constant2 : Constant  Value=uint8(1)
  Constant3 : Constant  Value=HVSR_bIsoResShieldCal
  Constant4 : Constant  Value=uint8(4)
  Constant5 : Constant  Value=HVSR_uBattVoltRngLo_C  OutDataTypeStr=single
  Constant6 : Constant  Value=boolean(1)
  Constant7 : Constant  Value=HVSR_uBattVoltRngHi_C  OutDataTypeStr=single
  Constant8 : Constant  Value=uint8(3)
  Constant9 : Constant  Value=uint8(5)
  Logical Operator : Logic  Operator=OR  Inputs=6  AllPortsSameDT=off  OutDataTypeStr=boolean
  Logical Operator1 : Logic  Operator=OR  AllPortsSameDT=off  OutDataTypeStr=boolean
  Logical Operator2 : Logic  Operator=OR  Inputs=4  AllPortsSameDT=off  OutDataTypeStr=boolean
  Logical Operator3 : Logic  Operator=OR  Inputs=4  AllPortsSameDT=off  OutDataTypeStr=boolean
  Relational Operator{,1,4..6,9..10,12,14} (9 alike) : RelationalOperator  Operator===  OutDataTypeStr=boolean  RndMeth=Simplest
  Relational Operator2 : RelationalOperator  Operator=>  OutDataTypeStr=boolean  RndMeth=Simplest
  Relational Operator3 : RelationalOperator  Operator=<  OutDataTypeStr=boolean  RndMeth=Simplest
  Switch : Switch  Criteria=u2 ~= 0
  TONV_100msTimeDebounce : Subsystem  TreatAsAtomicUnit=on  RTWFcnName=TONV_100msTimeDebounce  RTWFileName=SrvLib
  HVSR_IsoChieldCmd : Outport
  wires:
  COMR_bIsoResCalShieldCmd/1 -> Logical Operator/1
  BCMR_bDChrgIsoStopCmd/1 -> Logical Operator/2
  Logical Operator/1 -> Switch/3  "HVSR_bIsoResCalShieldCmd"
  Switch/1 -> HVSR_IsoChieldCmd/1
  Constant6/1 -> Switch/1
  Constant3/1 -> Switch/2
  TONV_100msTimeDebounce/1(y) -> Logical Operator/3
  Constant4/1 -> Relational Operator/2
  DSMR_stFaultRank/1 -> Relational Operator/1
  Constant1/1 -> TONV_100msTimeDebounce/2(T)
  Relational Operator/1 -> TONV_100msTimeDebounce/1(u)
  BSPR_uBattVolt/1 -> Relational Operator2/1, Relational Operator3/1
  Constant5/1 -> Relational Operator3/2
  Constant7/1 -> Relational Operator2/2
  Relational Operator2/1 -> Logical Operator1/1
  Relational Operator3/1 -> Logical Operator1/2
  Logical Operator1/1 -> Logical Operator/4
  Constant2/1 -> Relational Operator1/2
  Logical Operator2/1 -> Logical Operator/5
  Constant16/1 -> Relational Operator9/2
  Constant17/1 -> Relational Operator10/2
  BCCR_stBmsDChrgCtrMode/1 -> Relational Operator14/1, Relational Operator12/1, Relational Operator10/1, Relational Operator9/1
  Constant13/1 -> Relational Operator12/2
  Constant15/1 -> Relational Operator14/2
  Relational Operator9/1 -> Logical Operator3/1
  Relational Operator10/1 -> Logical Operator3/2
  Relational Operator12/1 -> Logical Operator3/3
  Logical Operator3/1 -> Logical Operator/6
  Relational Operator1/1 -> Logical Operator2/1
  Relational Operator4/1 -> Logical Operator2/2
  Constant8/1 -> Relational Operator4/2
  Constant9/1 -> Relational Operator5/2
  Relational Operator5/1 -> Logical Operator2/3
  Constant10/1 -> Relational Operator6/2
  BCCR_stBmsCtrMode/1 -> Relational Operator6/1, Relational Operator5/1, Relational Operator4/1, Relational Operator1/1
  Relational Operator6/1 -> Logical Operator2/4
  Relational Operator14/1 -> Logical Operator3/4

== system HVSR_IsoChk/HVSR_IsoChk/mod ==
  In1 : Inport
  Constant3 : Constant  Value=HVSR_stBMSModeLvl_C
  Constant4 : Constant  Value=enmBmsMode.STANDBY  OutDataTypeStr=Enum:enmBmsMode
  Data Type Conversion : DataTypeConversion  OutDataTypeStr=uint8
  Data Type Conversion1 : DataTypeConversion  OutDataTypeStr=uint8
  Logical Operator : Logic  AllPortsSameDT=off  OutDataTypeStr=boolean
  Relational Operator : RelationalOperator  OutDataTypeStr=boolean  RndMeth=Simplest
  Relational Operator1 : RelationalOperator  Operator=<=  OutDataTypeStr=boolean  RndMeth=Simplest
  Out1 : Outport
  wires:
  In1/1 -> Relational Operator/1, Relational Operator1/1
  Relational Operator/1 -> Logical Operator/1
  Relational Operator1/1 -> Logical Operator/2
  Constant3/1 -> Data Type Conversion1/1
  Constant4/1 -> Data Type Conversion/1
  Logical Operator/1 -> Out1/1
  Data Type Conversion/1 -> Relational Operator/2
  Data Type Conversion1/1 -> Relational Operator1/2

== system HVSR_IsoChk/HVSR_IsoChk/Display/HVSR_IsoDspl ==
  In1 : Inport
  In3 : Inport  Port=2
  Compare To Zero : simulink/Logic and Bit Operations/Compare To Zero  relop===  OutDataTypeStr=boolean
  Constant : Constant  Value=single(7777)
  Constant6 : Constant  Value=single(0)
  Constant8 : Constant  Value=HVSR_tiTaskTime_C
  Constant9 : Constant  Value=HVSR_ResFirstCtrlSw_C
  Relational Operator : RelationalOperator  Operator===  OutDataTypeStr=boolean  RndMeth=Simplest
  Switch10 : Switch  Criteria=u2 > Threshold
  Switch11 : Switch  Criteria=u2 > Threshold
  Switch12 : Switch  Criteria=u2 > Threshold
  Timer2 : Subsystem
  HVSR_resIso : Outport
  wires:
  Constant8/1 -> Timer2/2(Ts)
  Timer2/1(Timer) -> Compare To Zero/1
  Compare To Zero/1 -> Switch11/2
  In3/1 -> Switch12/3, Switch10/3, Switch11/3, Relational Operator/1  "HVSR_rInsResVal"
  Constant6/1 -> Relational Operator/2
  Relational Operator/1 -> Switch10/2  "HVSR_bInsResValZero"
  Switch12/1 -> HVSR_resIso/1
  Switch10/1 -> Switch11/1
  Switch11/1 -> Switch12/1  "HVSR_resIso"
  Constant9/1 -> Switch12/2
  In1/1 -> Timer2/1(En)
  Constant/1 -> Switch10/1

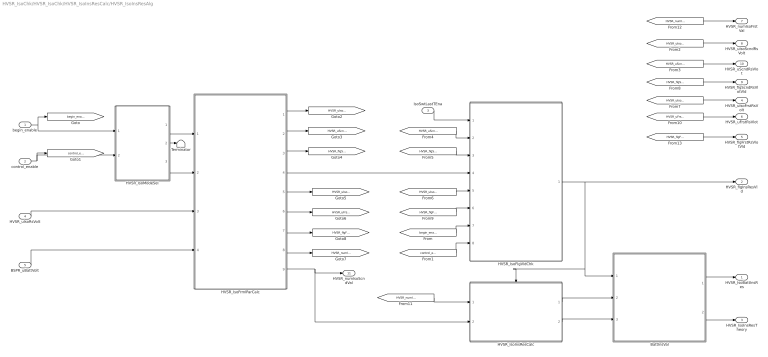
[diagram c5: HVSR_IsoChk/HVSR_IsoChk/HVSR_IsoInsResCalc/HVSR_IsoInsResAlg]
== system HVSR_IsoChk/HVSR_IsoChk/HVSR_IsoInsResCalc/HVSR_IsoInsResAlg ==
  begin_enable : Inport
  control_enable : Inport  Port=2
  IsoSwtLastTEna : Inport  Port=3
  HVSR_uIsoRsVolt : Inport  Port=4
  BSPR_uBattVolt : Inport  Port=5
  BattInsVal : Subsystem
  HVSR_IsoFlgVldChk : Subsystem  Description=Check whether the input voltage is zero, and check whether the total input voltage meets the total voltage requirement of the battery pack.
  HVSR_IsoFrmlParCalc : Subsystem
  HVSR_IsoInsResCalc : Subsystem  Description=Calculate the resistance of insulation resistance
  HVSR_IsoModeSel : Subsystem
  Terminator : Terminator
  HVSR_IsoBattInsRes : Outport
  HVSR_flgInsResVld : Outport  Port=2
  HVSR_IsoInsResTheory : Outport  Port=3
  HVSR_uIsoFrstRsVolt : Outport  Port=4
  HVSR_flgFrstRsVlotVld : Outport  Port=5
  HVSR_uFrstRsVlot : Outport  Port=6  InitialOutput=0
  HVSR_numIsoFrstVal : Outport  Port=7
  HVSR_uIsoScndRsVolt : Outport  Port=8
  HVSR_flgScndRsVlotVld : Outport  Port=9
  HVSR_uScndRsVlot : Outport  Port=10  InitialOutput=0
  HVSR_numIsoScndVal : Outport  Port=11
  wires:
  IsoSwtLastTEna/1 -> HVSR_IsoFlgVldChk/1(IsoSwtLastTEna)
  HVSR_IsoFlgVldChk/1(HVSR_flgInsResVld) -> HVSR_flgInsResVld/1, BattInsVal/1(HVSR_flgInsResVld), HVSR_IsoInsResCalc/Enable
  begin_enable/1 -> HVSR_IsoModeSel/1(begin_enable), [begin_enable]
  control_enable/1 -> HVSR_IsoModeSel/2(control_enable), [control_enable]
  BattInsVal/1(HVSR_IsoBattInsRes) -> HVSR_IsoBattInsRes/1
  BattInsVal/2(HVSR_IsoInsResTheory) -> HVSR_IsoInsResTheory/1
  [begin_enable] -> HVSR_IsoFlgVldChk/7(begin_enable)
  [control_enable] -> HVSR_IsoFlgVldChk/8(control_enable)
  HVSR_IsoInsResCalc/1(HVSR_resBattInsRes) -> BattInsVal/2(HVSR_resBattInsRes)
  HVSR_IsoInsResCalc/2(HVSR_resIsoTheory) -> BattInsVal/3(HVSR_resIsoTheory)
  HVSR_uIsoRsVolt/1 -> HVSR_IsoFrmlParCalc/3(HVSR_uIsoRsVolt)
  BSPR_uBattVolt/1 -> HVSR_IsoFrmlParCalc/4(BSPR_uBattVolt)
  HVSR_IsoFrmlParCalc/1(HVSR_uIsoScndRsVolt) -> [HVSR_uIsoScndRsVolt]
  HVSR_IsoFrmlParCalc/2(HVSR_uScndRsVlot) -> [HVSR_uScndRsVlot]
  HVSR_IsoFrmlParCalc/3(HVSR_flgScndRsVlotVld) -> [HVSR_flgScndRsVlotVld]
  HVSR_IsoFrmlParCalc/9(HVSR_numIsoScndVal) -> HVSR_numIsoScndVal/1, HVSR_IsoInsResCalc/2(HVSR_numIsoScndVal)
  HVSR_IsoFrmlParCalc/5(HVSR_uIsoFrstRsVolt) -> [HVSR_uIsoFrstRsVolt]
  HVSR_IsoFrmlParCalc/6(HVSR_uFrstRsVlot) -> [HVSR_uFrstRsVlot]
  HVSR_IsoFrmlParCalc/7(HVSR_flgFrstRsVlotVld) -> [HVSR_flgFrstRsVlotVld]
  HVSR_IsoFrmlParCalc/8(HVSR_numIsoFrstVal) -> [HVSR_numIsoFrstVal]
  HVSR_IsoModeSel/2(Out3) -> Terminator/1
  HVSR_IsoModeSel/3(control_on) -> HVSR_IsoFrmlParCalc/2(control_on)
  HVSR_IsoFrmlParCalc/4(HVSR_uBattVolt) -> HVSR_IsoFlgVldChk/4(HVSR_uBattVolt)
  [HVSR_uIsoScndRsVolt] -> HVSR_uIsoScndRsVolt/1
  [HVSR_uScndRsVlot] -> HVSR_uScndRsVlot/1
  [HVSR_uScndRsVlot] -> HVSR_IsoFlgVldChk/2(HVSR_uScndRsVlot)
  [HVSR_flgScndRsVlotVld] -> HVSR_IsoFlgVldChk/3(HVSR_flgScndRsVlotVld)
  [HVSR_uIsoFrstRsVolt] -> HVSR_IsoFlgVldChk/5(HVSR_uFrstRsVlot)
  [HVSR_uIsoFrstRsVolt] -> HVSR_uIsoFrstRsVolt/1
  [HVSR_flgScndRsVlotVld] -> HVSR_flgScndRsVlotVld/1
  [HVSR_flgFrstRsVlotVld] -> HVSR_IsoFlgVldChk/6(HVSR_flgFrstRsVlotVld)
  [HVSR_uFrstRsVlot] -> HVSR_uFrstRsVlot/1
  [HVSR_numIsoFrstVal] -> HVSR_IsoInsResCalc/1(HVSR_numIsoFrstVal)
  [HVSR_numIsoFrstVal] -> HVSR_numIsoFrstVal/1
  [HVSR_flgFrstRsVlotVld] -> HVSR_flgFrstRsVlotVld/1
  HVSR_IsoModeSel/1(begin_on) -> HVSR_IsoFrmlParCalc/1(begin_on)

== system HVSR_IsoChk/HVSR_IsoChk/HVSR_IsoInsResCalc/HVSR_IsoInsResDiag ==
  HVSR_IsoBattInsRes : Inport
  Compare To Zero : simulink/Logic and Bit Operations/Compare To Zero  relop=~=  OutDataTypeStr=boolean
  Constant10 : Constant  Value=HVSR_resIsoFaultLvl1Thres_C
  Constant6 : Constant  Value=HVSR_resIsoFaultLvl2Thres_C
  Constant9 : Constant  Value=HVSR_resIsoFaultLvl2Thres_C
  Delay : Delay  DelayLength=1  InitialCondition=0
  Delay2 : Delay  DelayLength=1  InitialCondition=0
  Logical Operator : Logic  AllPortsSameDT=off  OutDataTypeStr=boolean
  Logical Operator1 : Logic  AllPortsSameDT=off  OutDataTypeStr=boolean
  Relational Operator : RelationalOperator  OutDataTypeStr=boolean  RndMeth=Simplest
  Relational Operator3 : RelationalOperator  Operator=<  OutDataTypeStr=boolean  RndMeth=Simplest
  Relational Operator4 : RelationalOperator  OutDataTypeStr=boolean  RndMeth=Simplest
  BattIsolationFaultLvl2 : Outport
  BattIsolationFaultLvl1 : Outport  Port=2
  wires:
  HVSR_IsoBattInsRes/1 -> Delay2/1, Delay/1
  Logical Operator/1 -> BattIsolationFaultLvl2/1
  Relational Operator/1 -> Logical Operator/1
  Compare To Zero/1 -> Logical Operator/2
  Delay/1 -> Compare To Zero/1, Relational Operator/2
  Delay2/1 -> Relational Operator4/2, Relational Operator3/2
  Logical Operator1/1 -> BattIsolationFaultLvl1/1
  Constant6/1 -> Relational Operator/1
  Constant9/1 -> Relational Operator3/1
  Constant10/1 -> Relational Operator4/1
  Relational Operator3/1 -> Logical Operator1/1
  Relational Operator4/1 -> Logical Operator1/2

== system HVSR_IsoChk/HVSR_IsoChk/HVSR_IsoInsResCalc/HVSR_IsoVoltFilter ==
  BSPR_uIsoPosVolt : Inport
  Constant1 : Constant  Value=HVSR_uIsoPosVoltFilter_C  VectorParams1D=off
  K_Lowpass2 : Subsystem  TreatAsAtomicUnit=on  RTWFcnName=K_Lowpass  RTWFileName=SrvLib
  HVSR_uIsoRsVolt : Outport
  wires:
  K_Lowpass2/1(y) -> HVSR_uIsoRsVolt/1
  Constant1/1 -> K_Lowpass2/1(k)
  BSPR_uIsoPosVolt/1 -> K_Lowpass2/2(u)

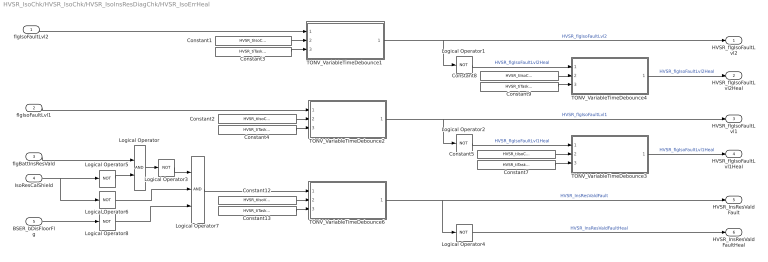
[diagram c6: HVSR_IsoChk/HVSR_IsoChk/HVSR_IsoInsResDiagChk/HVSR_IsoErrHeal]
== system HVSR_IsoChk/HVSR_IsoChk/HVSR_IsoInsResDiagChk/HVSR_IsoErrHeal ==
  flgIsoFaultLvl2 : Inport
  flgIsoFaultLvl1 : Inport  Port=2
  flgBattInsResVald : Inport  Port=3
  IsoResCalShield : Inport  Port=4
  BSER_bDisFloorFlg : Inport  Port=5
  Constant{1..2,5,8} (4 alike) : Constant  Value=HVSR_tiIsoChkDebounce_C
  Constant12 : Constant  Value=HVSR_tiIsoVldChkDebounce_C
  Constant{3..4,7,9,13} (5 alike) : Constant  Value=HVSR_tiTaskTime_C
  Logical Operator : Logic  AllPortsSameDT=off  OutDataTypeStr=boolean
  Logical Operator{1..6,8} (7 alike) : Logic  Operator=NOT  AllPortsSameDT=off  OutDataTypeStr=boolean
  Logical Operator7 : Logic  Inputs=3  AllPortsSameDT=off  OutDataTypeStr=boolean
  TONV_VariableTimeDebounce1 : Subsystem  TreatAsAtomicUnit=on  RTWFcnName=TONV_VariableTimeDebounce  RTWFileName=SrvLib
  TONV_VariableTimeDebounce2 : Subsystem  TreatAsAtomicUnit=on  RTWFcnName=TONV_VariableTimeDebounce  RTWFileName=SrvLib
  TONV_VariableTimeDebounce3 : Subsystem  TreatAsAtomicUnit=on  RTWFcnName=TONV_VariableTimeDebounce  RTWFileName=SrvLib
  TONV_VariableTimeDebounce4 : Subsystem  TreatAsAtomicUnit=on  RTWFcnName=TONV_VariableTimeDebounce  RTWFileName=SrvLib
  TONV_VariableTimeDebounce6 : Subsystem  TreatAsAtomicUnit=on  RTWFcnName=TONV_VariableTimeDebounce  RTWFileName=SrvLib
  HVSR_flgIsoFaultLvl2 : Outport
  HVSR_flgIsoFaultLvl2Heal : Outport  Port=2
  HVSR_flgIsoFaultLvl1 : Outport  Port=3
  HVSR_flgIsoFaultLvl1Heal : Outport  Port=4
  HVSR_InsResValdFault : Outport  Port=5
  HVSR_InsResValdFaultHeal : Outport  Port=6
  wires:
  flgIsoFaultLvl2/1 -> TONV_VariableTimeDebounce1/1(u)
  TONV_VariableTimeDebounce1/1(y) -> HVSR_flgIsoFaultLvl2/1, Logical Operator1/1  "HVSR_flgIsoFaultLvl2"
  flgIsoFaultLvl1/1 -> TONV_VariableTimeDebounce2/1(u)
  TONV_VariableTimeDebounce2/1(y) -> HVSR_flgIsoFaultLvl1/1, Logical Operator2/1  "HVSR_flgIsoFaultLvl1"
  Constant2/1 -> TONV_VariableTimeDebounce2/2(T)
  Constant4/1 -> TONV_VariableTimeDebounce2/3(dT)
  Constant1/1 -> TONV_VariableTimeDebounce1/2(T)
  Constant3/1 -> TONV_VariableTimeDebounce1/3(dT)
  Constant5/1 -> TONV_VariableTimeDebounce3/2(T)
  Constant7/1 -> TONV_VariableTimeDebounce3/3(dT)
  Logical Operator2/1 -> TONV_VariableTimeDebounce3/1(u)  "HVSR_flgIsoFaultLvl1Heal"
  Constant8/1 -> TONV_VariableTimeDebounce4/2(T)
  Constant9/1 -> TONV_VariableTimeDebounce4/3(dT)
  Logical Operator1/1 -> TONV_VariableTimeDebounce4/1(u)  "HVSR_flgIsoFaultLvl2Heal"
  flgBattInsResVald/1 -> Logical Operator/1
  Logical Operator3/1 -> Logical Operator7/1
  Constant12/1 -> TONV_VariableTimeDebounce6/2(T)
  Constant13/1 -> TONV_VariableTimeDebounce6/3(dT)
  TONV_VariableTimeDebounce6/1(y) -> HVSR_InsResValdFault/1, Logical Operator4/1  "HVSR_InsResValdFault"
  TONV_VariableTimeDebounce4/1(y) -> HVSR_flgIsoFaultLvl2Heal/1  "HVSR_flgIsoFaultLvl2Heal"
  TONV_VariableTimeDebounce3/1(y) -> HVSR_flgIsoFaultLvl1Heal/1  "HVSR_flgIsoFaultLvl1Heal"
  IsoResCalShield/1 -> Logical Operator6/1, Logical Operator5/1
  Logical Operator5/1 -> Logical Operator/2
  Logical Operator/1 -> Logical Operator3/1
  Logical Operator6/1 -> Logical Operator7/2
  Logical Operator7/1 -> TONV_VariableTimeDebounce6/1(u)
  Logical Operator4/1 -> HVSR_InsResValdFaultHeal/1  "HVSR_InsResValdFaultHeal"
  BSER_bDisFloorFlg/1 -> Logical Operator8/1
  Logical Operator8/1 -> Logical Operator7/3
